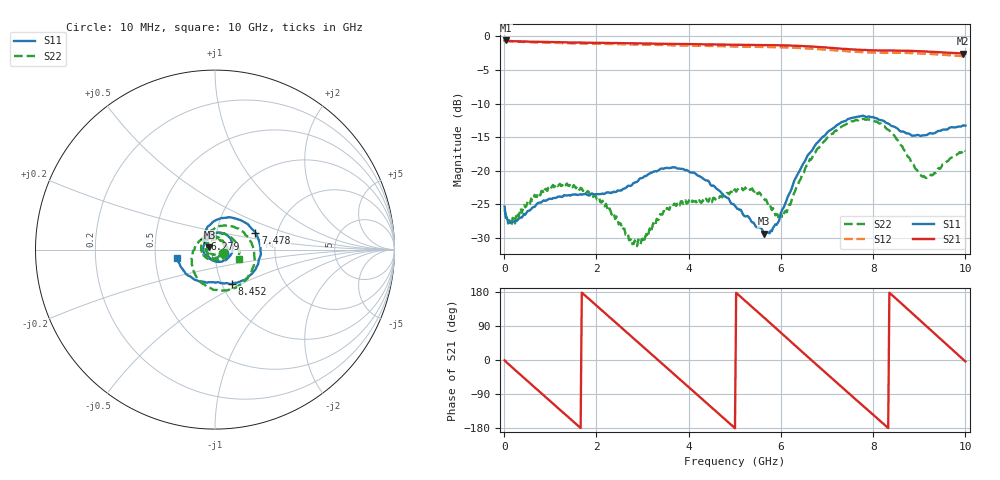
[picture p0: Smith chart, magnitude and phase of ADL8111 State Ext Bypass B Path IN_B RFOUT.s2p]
! Analog Devices Inc.
! Device:  ADL8111
! Description: Bypass Amplifier
! Frequency:  0.00 -  8.00 GHz
! Package:28-Lead Lead Frame Chip Scale Package[LFCSP] 6mm by 6mm
! Conditions:	Vdd = 5.0 V
!		State: External Bypass B
!		Path:  IN_B (Port1) to RFOUT (Port 2)
!		Idq = 70mA
!		Pin = -10 dBm
!		Temp = +25 C (baseplate temperature)
! Freq(Hz)	S11a(dB)	S11p(deg)	S21a(dB)	S21p(deg)	S12a(dB)	S12p(deg)	S22a(dB)	S22p(deg)
# Hz S  dB  R 50
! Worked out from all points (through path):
!   401 points, 10 MHz to 10 GHz, reference 50 ohm
!   highest |S21| = -0.62 dB at 34.98 MHz (marker M1); lowest = -2.6 dB at 9.95 GHz (marker M2)
!   group delay of S21, straight-line fit = 300 ps
!   lowest |S11| = -29.4 dB at 5.629 GHz (marker M3), VSWR 1.07, Z = 47 + j1.29 ohm
!   |S11| at or under -10 dB: start of sweep to end of sweep
!   |S22| runs from -31.2 to -12.3 dB; largest |S21 - S12| = 0.034
!   S11 on the Smith chart (normalised r, x): 10 MHz: 1.10, -0.05; 6.279 GHz: 0.88, +0.10; 7.478 GHz: 1.54, +0.31; 8.452 GHz: 1.12, -0.45; 10 GHz: 0.65, -0.06
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1e7  -25.32 -23.1  -0.64 -0.8  -0.62 -0.7  -25.87 -24.3
3.4975e7  -26.97 -18.4  -0.62 -4.1  -0.67 -4.0  -26.57 -16.0
4.84525e8  -26.24 -82.7  -0.79 -53.1  -0.85 -53.1  -25.18 -99.4
8.34175e8  -24.50 -124.7  -0.83 -90.9  -0.93 -90.9  -23.02 -156.6
1.3087e9  -23.61 -170.0  -0.91 -141.9  -1.01 -141.9  -22.20 140.0
1.683325e9  -23.54 163.6  -0.94 177.8  -1.07 177.8  -22.64 90.4
2.132875e9  -23.39 137.4  -0.98 129.5  -1.12 129.5  -24.43 29.1
2.5075e9  -22.94 120.6  -1.02 89.2  -1.16 89.2  -27.81 -28.2
2.982025e9  -21.10 94.7  -1.06 38.1  -1.23 38.1  -30.15 -134.7
3.35665e9  -19.88 64.3  -1.11 -2.3  -1.28 -2.2  -27.18 155.4
3.8062e9  -19.68 22.3  -1.15 -50.7  -1.35 -50.6  -25.14 102.6
4.180825e9  -20.62 -15.8  -1.18 -90.9  -1.40 -91.0  -24.88 66.8
5.005e9  -25.23 -126.1  -1.26 -179.9  -1.50 -179.9  -22.75 -3.1
5.629375e9  -29.36 156.2  -1.32 112.5  -1.58 112.6  -24.14 -67.5
6.278725e9  -21.69 135.3  -1.38 41.5  -1.70 41.6  -23.47 147.7
6.678325e9  -16.95 100.3  -1.53 -2.2  -1.84 -2.1  -18.06 83.1
7.477525e9  -12.25 22.7  -1.93 -88.6  -2.23 -88.5  -12.81 -15.8
8.35165e9  -13.06 -55.9  -2.10 177.7  -2.42 177.9  -14.01 -113.0
8.45155e9  -13.43 -63.6  -2.12 166.7  -2.44 166.9  -14.71 -124.2
9.175825e9  -14.66 -101.2  -2.27 87.0  -2.61 87.2  -20.90 105.3
9.95005e9  -13.26 -163.8  -2.58 1.5  -2.95 1.7  -16.84 -15.9
1e10  -13.29 -167.7  -2.58 -3.9  -2.97 -3.7  -17.06 -21.0
